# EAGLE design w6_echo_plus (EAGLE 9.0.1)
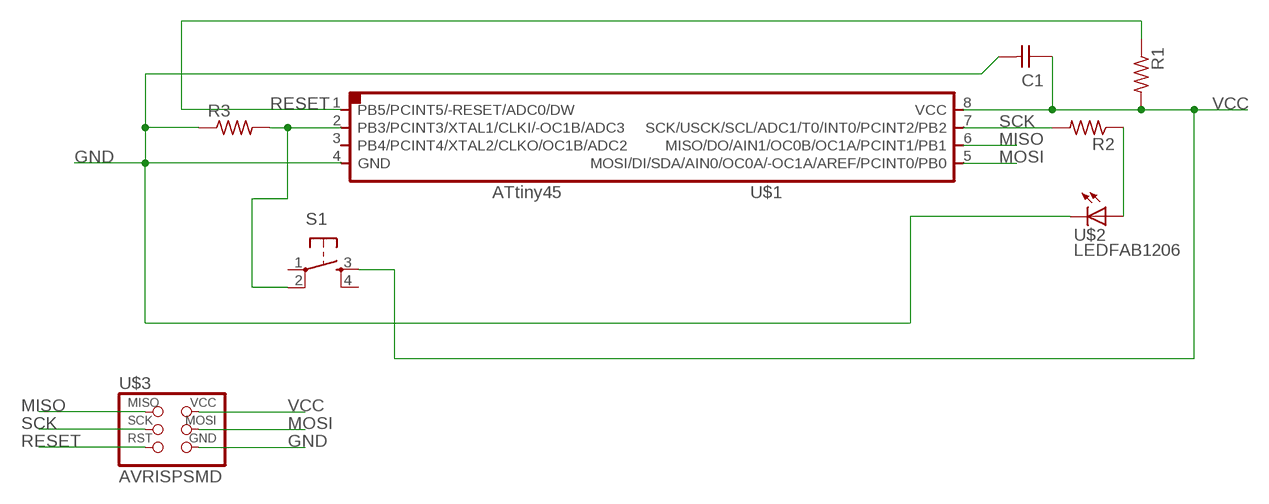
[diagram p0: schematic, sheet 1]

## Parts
C1  CAP-UNPOLARIZEDFAB  [C1206FAB]
R1  RES-US1206FAB  [R1206FAB]
R2  RES-US1206FAB  [R1206FAB]
R3  RES-US1206FAB  [R1206FAB]
S1  6MM_SWITCH6MM_SWITCH  [6MM_SWITCH]
U$1  ATTINY45SI  [SOIC8]
U$2  LEDFAB1206  [LED1206FAB]
U$3  AVRISPSMD  [2X03SMD]

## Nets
GND: C1.2 R3.1 U$1.4(GND) U$2.2(C) U$3.6(GND)
MISO: U$1.6(MISO/DO/AIN1/OC0B/OC1A/PCINT1/PB1) U$3.1(MISO)
MOSI: U$1.5(MOSI/DI/SDA/AIN0/OC0A/-OC1A/AREF/PCINT0/PB0) U$3.4(MOSI)
N$1: R3.2 S1.2(P1) U$1.2(PB3/PCINT3/XTAL1/CLKI/-OC1B/ADC3)
N$4: R2.1 U$2.1(A)
RESET: R1.1 U$1.1(PB5/PCINT5/-RESET/ADC0/DW) U$3.5(RST)
SCK: R2.2 U$1.7(SCK/USCK/SCL/ADC1/T0/INT0/PCINT2/PB2) U$3.3(SCK)
VCC: C1.1 R1.2 S1.3(S) U$1.8(VCC) U$3.2(VCC)
Unconnected: S1.1(P) S1.4(S1) U$1.3(PB4/PCINT4/XTAL2/CLKO/OC1B/ADC2)

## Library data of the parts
C1 = fab:CAP-UNPOLARIZED
R1-R3 = fab:RES-US: Resistor (US Symbol)
S1 = fab:6MM_SWITCH: OMRON SWITCH
U$1 = fab:ATTINY45
U$2 = fab:LED: LED
U$3 = fab:AVRISP

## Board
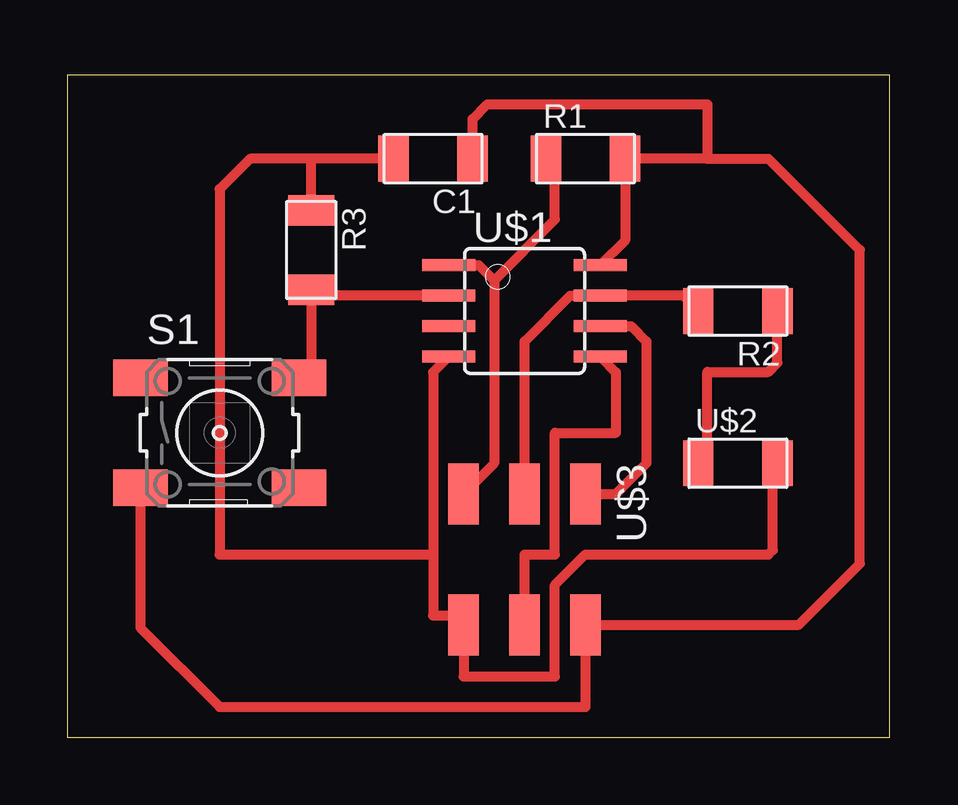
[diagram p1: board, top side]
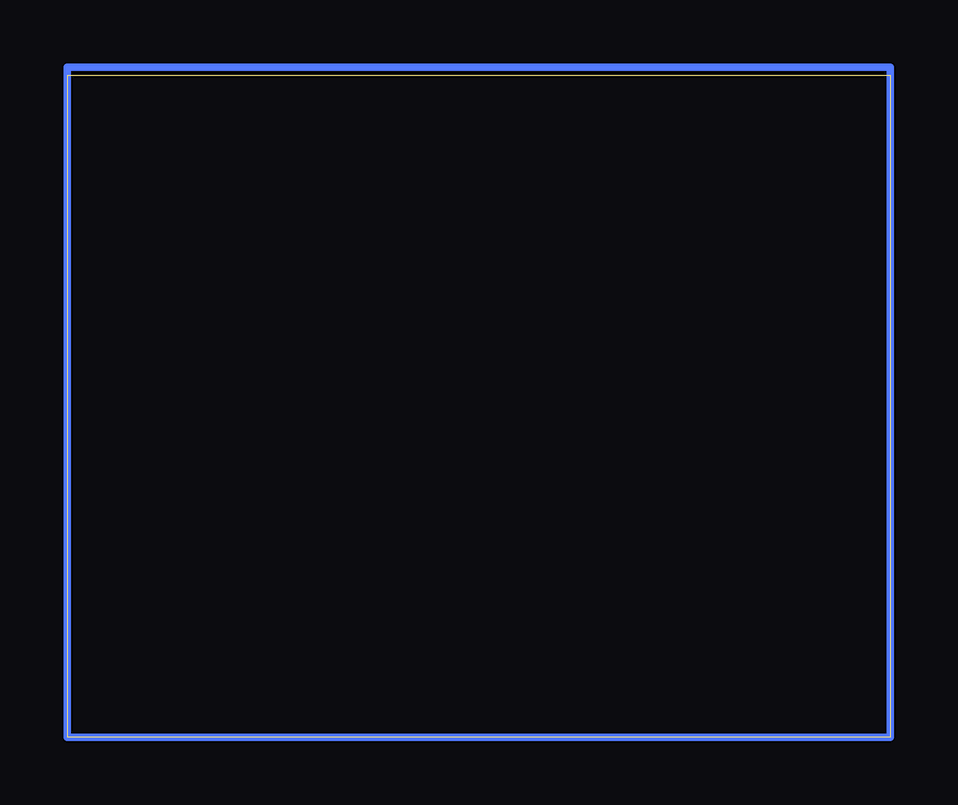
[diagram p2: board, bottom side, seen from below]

Size 34.27 x 27.61 mm. Coordinates in mm from the lower left corner, seen from the top.
Outline: 0,0 34.27,0 34.27,27.61 0,27.61 0,0
Copper layers (1*16): Top 0.035mm / dielectric 1.5mm / Bottom 0.035mm
Design rules "fabmodule": minimum track width 10mil, minimum drill 0.4mm, track to track 0.42mm, track to pad 0.42mm, pad to pad 0.42mm, via to via 0.42mm, smd to smd 0.42mm, copper to edge 40mil, drill to drill 0.8mm, minimum pad ring 10mil, minimum via ring 8mil, stop-mask expansion 4mil, vias tented up to drill 0mil, thermal gap 10mil

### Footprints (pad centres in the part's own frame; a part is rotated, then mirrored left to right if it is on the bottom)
C1206FAB = smd 1.27 x 1.905: 1 -1.651,0; 2 1.651,0
R1206FAB = smd 1.27 x 1.905: 1 -1.651,0; 2 1.651,0
6MM_SWITCH = smd 2.286 x 1.524: 1 -3.302,2.286; 2 3.302,2.286; 3 -3.302,-2.286; 4 3.302,-2.286
SOIC8 = smd 0.5 x 2.2: 1 -1.905,-3.154; 2 -0.645,-3.154; 3 0.625,-3.154; 4 1.895,-3.154; 5 1.905,3.154; 6 0.635,3.154; 7 -0.635,3.154; 8 -1.905,3.154
LED1206FAB = smd 1.27 x 1.905: 1 -1.651,0; 2 1.651,0
2X03SMD = smd 2.54 x 1.27: 1 -2.54,2.54; 2 2.92,2.54; 3 -2.54,0; 4 2.92,0; 5 -2.54,-2.54; 6 2.92,-2.54

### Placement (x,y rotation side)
C1  15.24,24.13 180 top
R1  21.59,24.13 0 top
R2  27.94,17.78 180 top
R3  10.16,20.32 270 top
S1  6.35,12.7 0 top
U$1  19.05,17.78 270 top
U$2  27.94,11.43 0 top
U$3  19.05,7.62 270 top

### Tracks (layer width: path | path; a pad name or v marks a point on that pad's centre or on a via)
GND
  Top 0.406: U$2.2 29.4,11.24 | 29.4,11.24 29.21,11.05 | U$1.4 15.24,15.23 15.24,7.62 | 15.24,7.62 15.24,5.08 16.13,5.08 U$3.6 16.51,2.54 20.32,2.54 20.32,6.35 21.59,7.62 29.21,7.62 29.4,7.81 29.4,11.24 | 15.24,7.62 10.16,7.62 6.35,7.62 6.35,22.86 7.62,24.13 10.16,24.13 | C1.2 10.16,24.13 | R3.1 10.16,24.13
MISO
  Top 0.406: U$3.1 22.86,10.16 24.13,11.43 24.13,16.51 23.5,17.14 U$1.6
MOSI
  Top 0.406: U$1.5 22.86,15.22 22.86,12.7 20.32,12.7 20.32,7.62 19.05,7.62 U$3.4
N$1
  Top 0.406: S1.2 10.16,15.49 R3.2 10.4,18.43 U$1.2
N$2
  Bottom 0.305: 0,27.94 0,0 34.29,0 34.29,27.94 0,27.94
N$4
  Top 0.406: U$2.1 26.67,11.81 26.67,15.24 29.21,15.24 29.59,15.62 R2.1
RESET
  Top 0.406: U$3.5 17.78,11.43 17.78,19.05 | U$1.1 17.14,19.69 17.78,19.05 | 17.78,19.05 20.32,21.59 20.32,23.75 R1.1
SCK
  Top 0.406: U$3.3 19.05,16.51 20.95,18.41 U$1.7 25.65,18.41 R2.2
VCC
  Top 0.406: 26.67,24.13 29.21,24.13 33.02,20.32 33.02,7.24 30.48,4.7 U$3.2 21.59,1.27 6.35,1.27 3.05,4.57 S1.3 | 26.67,24.13 R1.2 23.24,20.72 U$1.8 | C1.1 16.89,25.78 17.5,26.39 24.13,26.39 26.67,26.39 26.67,24.13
